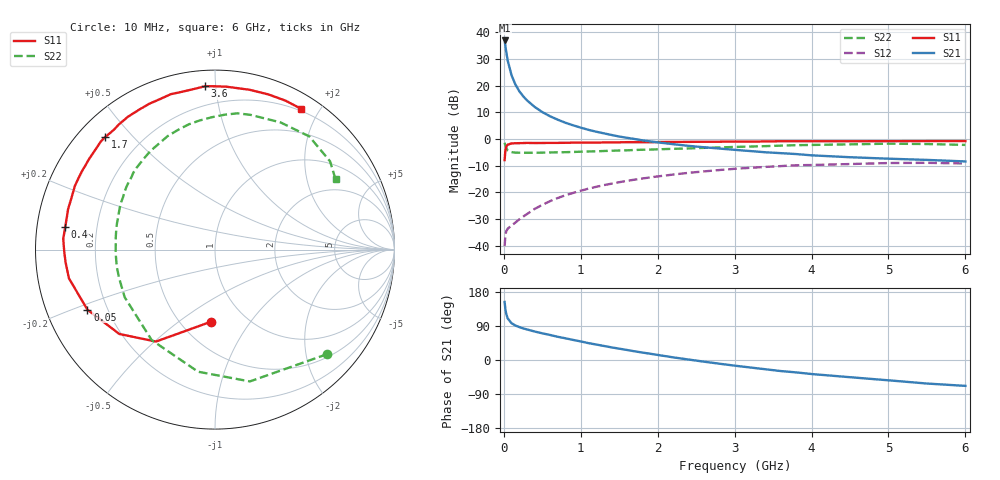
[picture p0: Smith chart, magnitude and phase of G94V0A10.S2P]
! SIEMENS Small Signal Semiconductors
! BFG235
! Si NPN RF Bipolar Junction Transistor in SOT223
! VCE = 4 V  IC = 100 mA
! Common Emitter S-Parameters:  July  1994
# GHz  S  MA  R  50
!  f  S11  S21  S12  S22
! GHz  MAG  ANG  MAG  ANG  MAG  ANG  MAG  ANG
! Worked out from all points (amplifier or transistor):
!   40 points, 10 MHz to 6 GHz, reference 50 ohm
!   highest |S21| = 37.0 dB at 10 MHz (marker M1)
!   |S21| within 3 dB of that: start of sweep to 24.88 MHz
!   unconditionally stable (mu >= 1): 467.8 MHz to 1.455 GHz
!   at 200 MHz: K = 0.77, MSG = 24.1 dB, |S12| = -30.1 dB
!   at 1.5 GHz: K = 1.00, MSG = 8.6 dB, |S12| = -16.2 dB
!   at 6 GHz: K = 0.90, MSG = 0.4 dB, |S12| = -9.2 dB
!   S11 on the Smith chart (normalised r, x): 10 MHz: 0.69, -0.67; 50 MHz: 0.13, -0.22; 400 MHz: 0.09, +0.08; 1.7 GHz: 0.08, +0.42; 3.6 GHz: 0.09, +0.94; 6 GHz: 0.17, +1.77
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0.01  0.4028 -93.3  70.88 153.2  0.0098 64.8  0.8542 -43.0
0.02  0.6089 -122.7  56.32 134.5  0.0153 49.8  0.7597 -75.2
0.03  0.7108 -138.6  44.46 122.6  0.0184 42.0  0.6869 -97.9
0.05  0.7858 -154.8  29.79 109.8  0.0209 33.4  0.6152 -125.0
0.1  0.8295 -168.9  15.79 97.2  0.0239 34.7  0.5689 -152.2
0.15  0.8357 -175.3  10.61 91.0  0.0272 40.6  0.5572 -163.6
0.2  0.8392 -178.6  7.943 87.0  0.0312 44.8  0.5556 -170.0
0.25  0.8434 178.3  6.401 83.5  0.035 48.8  0.5533 -174.4
0.3  0.8476 175.9  5.346 80.7  0.0392 51.6  0.5539 -178.0
0.4  0.8439 171.3  4.022 75.2  0.0489 54.9  0.5538 176.8
0.5  0.8452 167.5  3.213 70.4  0.0585 56.4  0.5574 172.6
0.6  0.849 164.6  2.684 66.1  0.0684 56.7  0.5611 168.7
0.7  0.8492 161.1  2.314 61.3  0.0784 56.5  0.5653 165.2
0.9  0.8575 155.5  1.814 53.0  0.0977 54.0  0.5736 159.1
1.1  0.8606 149.2  1.491 44.5  0.1177 51.0  0.5861 153.0
1.7  0.8765 134.4  1.004 22.9  0.1735 39.1  0.6252 136.7
2.2  0.885 123.2  0.803 7.0  0.2159 28.1  0.657 123.1
3.2  0.8983 101.6  0.597 -19.7  0.2892 5.0  0.7242 96.9
3.6  0.9118 93.5  0.545 -29.2  0.3116 -5.0  0.7538 85.8
4.5  0.9111 77.8  0.457 -45.4  0.3404 -24.9  0.7973 62.7
5.5  0.9182 64.7  0.407 -62.1  0.3586 -46.9  0.808 37.5
6  0.9195 58.6  0.381 -68.3  0.3486 -55.0  0.7776 30.3
